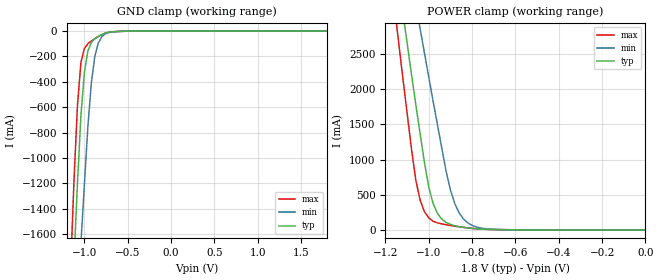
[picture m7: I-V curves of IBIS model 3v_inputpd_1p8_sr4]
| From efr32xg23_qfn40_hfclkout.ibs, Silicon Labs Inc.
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|   Model 3v_inputpd_1p8_sr4
[Model]  3v_inputpd_1p8_sr4
Model_type Input
C_comp   1.6300pF   1.4000pF   2.7000pF
[Temperature Range]   25.0000   0.1250k   -40.0000
[Pullup Reference]   1.8000V   1.6200V   1.9800V
[Pulldown Reference]   0.0V   0.0V   0.0V
[POWER Clamp Reference]   1.8000V   1.6200V   1.9800V
[GND Clamp Reference]   0.0V   0.0V   0.0V
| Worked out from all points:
|   GND clamp passes 1 mA (typ) near -0.52 V on its own axis
|   POWER clamp passes 1 mA (typ) near -0.53 V on its own axis
[GND_clamp]
|Voltage   I(typ)   I(min)   I(max)
-1.8V     -14.24A    -14.11A    -14.46A
-1.16V    -2.476A    -3.328A    -1.893A
-1.12V    -1.809A    -2.723A    -1.176A
-1.08V    -1.199A    -2.174A    -584.5mA
-1.04V    -665.3mA   -1.671A    -246.2mA
-1V       -325.1mA   -1.206A    -136.5mA
-960mV    -156.4mA   -753.1mA   -99.66mA
-920mV    -90.22mA   -408.8mA   -78.06mA
-880mV    -60.42mA   -199.9mA   -59.74mA
-840mV    -41.39mA   -94.68mA   -43.13mA
-640mV    -3.815mA   -4.276mA   -4.112mA
1.8V      40uA       35.07uA    46.81uA
[POWER_clamp]
|Voltage   I(typ)   I(min)   I(max)
-1.8V     20.85A     19.71A     22.07A
-1.16V    4.023A     5.096A     3.217A
-1.14V    3.56A      4.702A     2.691A
-1.1V     2.657A     3.938A     1.662A
-1.06V    1.785A     3.203A     711mA
-1.04V    1.371A     2.858A     425mA
-1V       612.4mA    2.171A     172.4mA
-980mV    375.2mA    1.828A     122.5mA
-900mV    79.41mA    567.6mA    63.76mA
-860mV    47.66mA    243.7mA    45.1mA
-820mV    29.36mA    101.5mA    29.71mA
0V        40uA       30.78uA    51.49uA
